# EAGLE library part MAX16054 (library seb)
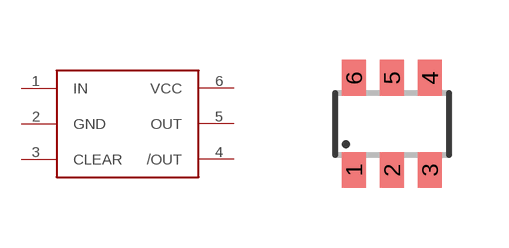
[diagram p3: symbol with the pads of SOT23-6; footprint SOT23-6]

Designator prefix IC

## MAX16054  [SOT23-6]
1  IN
2  GND
3  CLEAR
4  /OUT
5  OUT
6  VCC

## Footprint SOT23-6 (pad centres in mm)
Small Outline Transistor 6 lead
smd 0.6 x 0.9: 1 -0.95,-1.15; 2 0,-1.15; 3 0.95,-1.15; 4 0.95,1.15; 5 0,1.15; 6 -0.95,1.15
